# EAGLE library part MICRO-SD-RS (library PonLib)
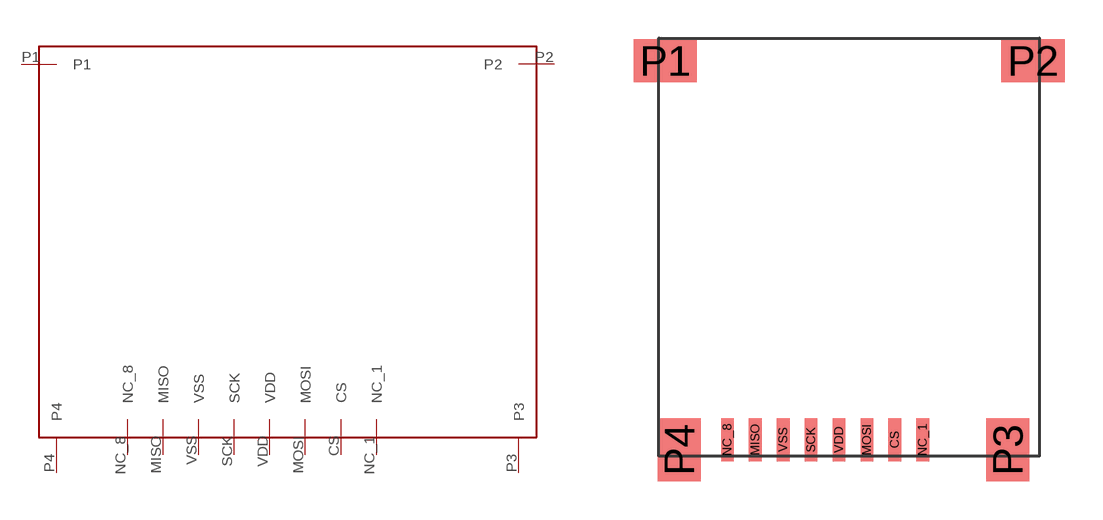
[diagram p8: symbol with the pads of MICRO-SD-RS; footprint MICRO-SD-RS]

Designator prefix -

## MICRO-SD-RS  [MICRO-SD-RS]
CS  CS
MISO  MISO
MOSI  MOSI
NC_1  NC_1
NC_8  NC_8
P1  P1
P2  P2
P3  P3
P4  P4
SCK  SCK
VDD  VDD
VSS  VSS

## Footprint MICRO-SD-RS (pad centres in mm)
smd 0.5 x 1.7: CS 1.8,-0.85; MISO -3.7,-0.85; MOSI 0.7,-0.85; NC_1 2.9,-0.85; NC_8 -4.8,-0.85; SCK -1.5,-0.85; VDD -0.4,-0.85; VSS -2.6,-0.85
smd 2.5 x 1.7: P1 -7.25,14.1; P2 7.25,14.1
smd 1.7 x 2.5: P3 6.25,-1.25; P4 -6.7,-1.25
